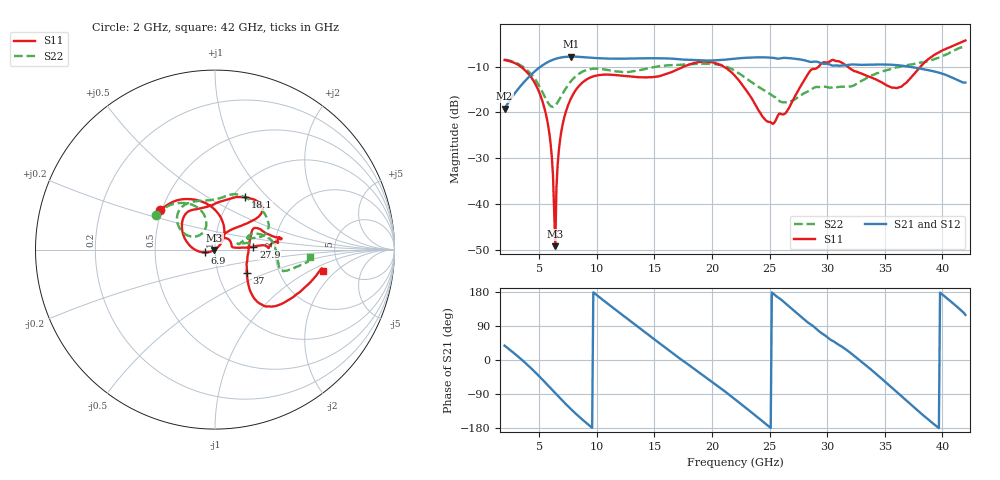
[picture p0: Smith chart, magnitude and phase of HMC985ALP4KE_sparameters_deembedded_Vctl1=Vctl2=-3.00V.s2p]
!s2p File: Measurements: S11, S21, S12, S22
# GHz S dB R 50.0
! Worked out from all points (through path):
!   401 points, 2 GHz to 42 GHz, reference 50 ohm
!   highest |S21| = -7.78 dB at 7.8 GHz (marker M1); lowest = -19.2 dB at 2 GHz (marker M2)
!   lowest |S11| = -49.2 dB at 6.4 GHz (marker M3), VSWR 1.01, Z = 49.7 - j0.148 ohm
!   |S11| at or under -10 dB: 3.405 GHz to 17.52 GHz (14.12 GHz wide, 135 % of centre); 21.04 GHz to 29.25 GHz (8.209 GHz wide, 32.7 % of centre); 31.79 GHz to 38.09 GHz (6.299 GHz wide, 18 % of centre)
!   |S22| runs from -18.8 to -5.5 dB; largest |S21 - S12| = 0.00044
!   S11 on the Smith chart (normalised r, x): 2 GHz: 0.49, +0.25; 6.9 GHz: 0.89, -0.03; 18.1 GHz: 1.15, +0.75; 27.9 GHz: 1.54, +0.05; 37 GHz: 1.37, -0.38; 42 GHz: 3.61, -1.37
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2  -8.53 144.4  -19.19 37.8  -19.20 37.8  -8.45 149.7
3.8  -10.85 108.1  -13.04 -7.7  -13.05 -7.7  -10.41 121.3
5.1  -16.20 73.2  -10.03 -45.9  -10.03 -45.9  -14.65 106.8
5.8  -23.17 51.2  -8.92 -68.3  -8.92 -68.3  -17.99 115.9
6.2  -33.80 39.9  -8.47 -81.2  -8.47 -81.2  -18.75 131.1
6.4  -49.24 -154.5  -8.29 -87.6  -8.29 -87.7  -18.45 139.1
6.9  -24.51 -164.3  -7.97 -103.6  -7.97 -103.6  -16.51 150.9
7.8  -16.73 169.8  -7.78 -130.8  -7.79 -130.9  -13.05 149.8
8.7  -13.59 150.4  -7.87 -155.9  -7.88 -155.9  -11.16 140.0
12.4  -12.00 117.0  -8.23 114.9  -8.23 114.8  -11.16 96.2
15.4  -12.09 93.1  -8.16 45.3  -8.16 45.3  -9.91 73.7
18.1  -9.45 59.7  -8.48 -15.5  -8.49 -15.5  -9.44 59.0
22  -11.99 38.2  -8.23 -103.7  -8.24 -103.7  -10.90 16.3
25.2  -22.38 60.8  -8.03 178.1  -8.03 178.1  -16.24 15.9
27.9  -13.38 4.4  -8.52 109.6  -8.52 109.6  -15.93 12.9
28.7  -10.53 1.9  -8.94 91.4  -8.95 91.4  -14.84 12.1
30.5  -8.50 9.3  -9.76 50.0  -9.76 50.0  -14.45 15.5
32.4  -10.99 22.0  -9.52 9.5  -9.52 9.5  -13.98 22.3
35.4  -14.32 7.5  -9.54 -67.3  -9.54 -67.4  -10.60 13.9
37  -13.14 -36.7  -9.94 -110.4  -9.95 -110.5  -9.62 5.0
39.5  -7.14 -46.1  -11.15 -174.9  -11.16 -175.0  -8.16 -17.1
42  -4.25 -11.1  -13.46 118.9  -13.47 118.8  -5.51 -4.6
